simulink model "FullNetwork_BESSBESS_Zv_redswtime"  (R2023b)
settings: Solver=ode15s  StartTime=0.0  StopTime=140  RelTol=1e-3
PreLoadFcn:
  | Ts=50e-6;
model workspace (MAT data in the model file):
  Cf1 = 0.02
  Cf2 = 0.02
  Kffi1 = 0.9
  Kffi2 = 0.9
  Kffi3 = 0.9
  Kffv1 = 1
  Kffv2 = 1
  Kffv3 = 1
  Ki_cc1 = 5.9
  Ki_cc2 = 5.9
  Ki_cc3 = 5.9
  Ki_q1 = 0.0001
  Ki_q2 = 0.0001
  Ki_q3 = 0.0001
  Ki_vc1 = 150
  Ki_vc2 = 150
  Ki_vc3 = 150
  Kp_cc1 = 0.015
  Kp_cc2 = 0.015
  Kp_vc1 = 5
  Kp_vc2 = 5
  Kp_vc3 = 5
  Lf1 = 4.75e-06
  Lf2 = 4.75e-06
  Rf1 = 0.0005
  Rf2 = 0.0005
  Rf3 = 0.0005
  Rv1 = 0.0003169
  Rv2 = 0.0003169
  Snom1 = 100000000
  Snom2 = 100000000
  Vdc1 = 2000
  Vdc2 = 2000
  Vdc3 = 2000
  Xv1 = 0.0009509
  Xv2 = 0.0009509
  fnom1 = 50
  fnom2 = 50
  mp1 = 6.25e-08
  mp2 = 6.25e-08
  nq1 = 4.69166666667e-07
  nq2 = 4.69166666667e-07
  tau1 = 0.001
  tau2 = 0.001
  tau3 = 0.001
  vnom1 = 690
  vnom2 = 690
  vnom3 = 690
undefined symbols (not defined in the file or in its folder): Armidale, DiscIntNeverNeededParam, find_system, Gunnedah, Innerell, Ion, Lithium, Morree, Narrabri, Tamworth
libraries: spsThreePhaseBreakerLib x41, spsThreePhaseVIMeasurementLib x16, simulink_extras x16, spsThreePhaseSeriesRLCLoadLib x14, spsabctodq0Lib x12, spsThreePhaseTransformerTwoWindingsLib x11, slpidlib x8, spsLoadFlowBusLib x8, spsThreePhasePISectionLineLib x8, powerlib_extras x7, spsFirstOrderFilterLib x6, simulink x5
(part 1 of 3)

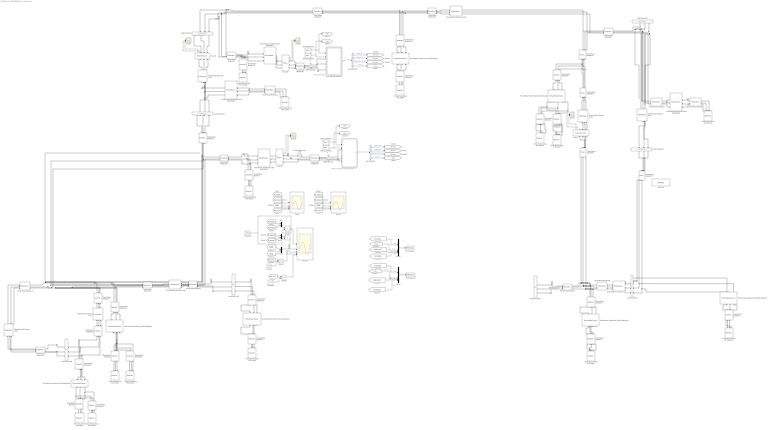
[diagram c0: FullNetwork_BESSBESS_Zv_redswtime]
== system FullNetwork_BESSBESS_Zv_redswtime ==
  note: Ts
  note: AC/DC conversion stage 80.0 MW
  note: Ts
  note: AC/DC conversion stage 80.0 MW
  B690 (690 V)1 : spsThreePhaseVIMeasurementLib/Three-Phase V-I Measurement  VoltageMeasurement=phase-to-ground  SetLabelV=on  LabelV=Vabc_B5751  Vpu=off  VpuLL=off  CurrentMeasurement=yes  SetLabelI=on  LabelI=Iabc_B5751  Ipu=off  Pbase=5*2e6/0.9  Vbase=575  OutputType=Complex  PhasorSimulation=off  PSBequivalent=0
  B690 (690 V)2 : spsThreePhaseVIMeasurementLib/Three-Phase V-I Measurement  VoltageMeasurement=phase-to-ground  SetLabelV=on  LabelV=Vabc_B5752  Vpu=off  VpuLL=off  CurrentMeasurement=yes  SetLabelI=on  LabelI=Iabc_B5752  Ipu=off  Pbase=5*2e6/0.9  Vbase=575  OutputType=Complex  PhasorSimulation=off  PSBequivalent=0
  B_grid1 : spsThreePhaseVIMeasurementLib/Three-Phase V-I Measurement  VoltageMeasurement=phase-to-ground  SetLabelV=off  LabelV=Vabc  Vpu=on  VpuLL=off  CurrentMeasurement=yes  SetLabelI=off  LabelI=Iabc  Ipu=on  Pbase=100e6  Vbase=132e3  OutputType=Complex  PhasorSimulation=off  PSBequivalent=0
  B_grid4 : spsThreePhaseVIMeasurementLib/Three-Phase V-I Measurement  VoltageMeasurement=phase-to-ground  SetLabelV=off  LabelV=Vabc  Vpu=on  VpuLL=off  CurrentMeasurement=yes  SetLabelI=off  LabelI=Iabc  Ipu=on  Pbase=100e6  Vbase=690  OutputType=Complex  PhasorSimulation=off  PSBequivalent=0
  B_grid5 : spsThreePhaseVIMeasurementLib/Three-Phase V-I Measurement  VoltageMeasurement=phase-to-ground  SetLabelV=off  LabelV=Vabc  Vpu=on  VpuLL=off  CurrentMeasurement=yes  SetLabelI=off  LabelI=Iabc  Ipu=on  Pbase=100e6  Vbase=690  OutputType=Complex  PhasorSimulation=off  PSBequivalent=0
  B_grid7 : spsThreePhaseVIMeasurementLib/Three-Phase V-I Measurement  VoltageMeasurement=phase-to-ground  SetLabelV=off  LabelV=Vabc  Vpu=on  VpuLL=off  CurrentMeasurement=yes  SetLabelI=off  LabelI=Iabc  Ipu=on  Pbase=100e6  Vbase=132e3  OutputType=Complex  PhasorSimulation=off  PSBequivalent=0
  Bus Selector1 : BusSelector  OutputSignals=Vabc_pcc,Iabc_pcc,Iabc_grid_conv_pu,Freq
  Bus Selector2 : BusSelector  OutputSignals=Vabc_pcc,Iabc_pcc,Iabc_grid_conv_pu,Freq
  Constant : Constant  Value=563
  Constant1 : Constant  Value=563
  Constant2 : Constant  Value=100e6
  Current Measurement2 : spsCurrentMeasurementLib/Current Measurement  PhasorSimulation=off  OutputType=Complex  PSBequivalent=0
  Divide{,1..3} (4 alike) : Product  Inputs=*/
  Grid forming inverter1 : Subsystem  LoadFcn=%find_system(gcs,'FollowLinks', 'on', 'LookUnderMasks', 'all');  mask(Grid forming inverter){Vnom=vnom1, fnom=fnom1, Pnom=Snom1, Lf=Lf1, Rf=Rf1, Cf=Cf1, Vdc_nom=Vdc1, Innerloops=Inner loops, Kp_cc=Kp_cc1, Ki_cc=Ki_cc1, Kffv=Kffv1, Kp_vc=Kp_vc1, Ki_vc=Ki_vc1, Kffi=Kffi1, Virtualimpedance=Virtual impedance, Rvir=Rv1, Lvir=Xv1, ControlType=Virtual Synchronous Machine, mp=mp1, nq=nq1, Ki_q=Ki_q1, tau=tau1, Ts=5e-5}
      mask prompts: Vnom "Grid-side converter nominal AC voltage (V):"; fnom "Grid frequency (Hz)"; Pnom "Nominal power (VA)"; Lf "Filter inductance (H)"; Rf "Filter resistance (Ω)"; Cf "Filter capacitor (F):"; Vdc_nom "Nominal DC bus voltage (V)"; Innerloops "Inner loops"; Kp_cc "Proportional gain of the current controller"; Ki_cc "Integral gain of the current controller"; Kffv "Voltage feed-forward"; Kp_vc "Proportional gain of the voltage controller"; Ki_vc "Integral gain of the voltage controller"; Kffi "Current feed-forward"; Virtualimpedance "Virtual impedance"; Rvir "Resistance of the virtual impedance"; Lvir "Inductance of the virtual impedance"; ControlType "Primary control"; mp "P - ω Droop coefficient"; nq "Q - V Droop coefficient"; Ki_q "Integral gain of the reactive power controller"; tau "Filter time constant (s)"; Ts "Sample time (s):"
      mask help: This block implements a model of a grid forming inverter with either droop or virtual synchronous generator control.
      mask init:
      | % Converters data
      | Q_filter=50;
      | 
      | % Controller data
      | Freq_filter=10000;   %Hz
      | Zeta_filter=0.707;
      | Mod_index_max=1.1;
      | T_speed=5;      %Speed reference time constant (s)
      | Iq_ref_limit_time_constant=0.3; %(s)
      | Current_reg_output_limit=1.1;   %(pu)
      | Var_reg_output_hi_limit=1.1;    %(pu)
      | Var_reg_output_low_limit=0.9;   %(pu)
      | Pitch_time_constant=0.01;       %(s)
      | Vf_limit=10;    %Field voltage limit (pu)
      | Freq_sawtooth=2000; %Hz, Boost converter
      | Freq_PWM=3000; %Hz, Inverter
      | Ts_snub=50e-6;  %Sample time to compute snubber resistance
  Grid forming inverter3 : Subsystem  LoadFcn=%find_system(gcs,'FollowLinks', 'on', 'LookUnderMasks', 'all');  mask(Grid forming inverter){Vnom=vnom2, fnom=fnom2, Pnom=Snom2, Lf=Lf2, Rf=Rf2, Cf=Cf2, Vdc_nom=Vdc2, Innerloops=Inner loops, Kp_cc=Kp_cc2, Ki_cc=Ki_cc2, Kffv=Kffv2, Kp_vc=Kp_vc2, Ki_vc=Ki_vc2, Kffi=Kffi2, Virtualimpedance=Virtual impedance, Rvir=Rv2, Lvir=Xv2, ControlType=Virtual Synchronous Machine, mp=mp2, nq=nq2, Ki_q=Ki_q2, tau=tau2, Ts=5e-5}
      mask prompts: Vnom "Grid-side converter nominal AC voltage (V):"; fnom "Grid frequency (Hz)"; Pnom "Nominal power (VA)"; Lf "Filter inductance (H)"; Rf "Filter resistance (Ω)"; Cf "Filter capacitor (F):"; Vdc_nom "Nominal DC bus voltage (V)"; Innerloops "Inner loops"; Kp_cc "Proportional gain of the current controller"; Ki_cc "Integral gain of the current controller"; Kffv "Voltage feed-forward"; Kp_vc "Proportional gain of the voltage controller"; Ki_vc "Integral gain of the voltage controller"; Kffi "Current feed-forward"; Virtualimpedance "Virtual impedance"; Rvir "Resistance of the virtual impedance"; Lvir "Inductance of the virtual impedance"; ControlType "Primary control"; mp "P - ω Droop coefficient"; nq "Q - V Droop coefficient"; Ki_q "Integral gain of the reactive power controller"; tau "Filter time constant (s)"; Ts "Sample time (s):"
      mask help: This block implements a model of a grid forming inverter with either droop or virtual synchronous generator control.
      mask init:
      | % Converters data
      | Q_filter=50;
      | 
      | % Controller data
      | Freq_filter=10000;   %Hz
      | Zeta_filter=0.707;
      | Mod_index_max=1.1;
      | T_speed=5;      %Speed reference time constant (s)
      | Iq_ref_limit_time_constant=0.3; %(s)
      | Current_reg_output_limit=1.1;   %(pu)
      | Var_reg_output_hi_limit=1.1;    %(pu)
      | Var_reg_output_low_limit=0.9;   %(pu)
      | Pitch_time_constant=0.01;       %(s)
      | Vf_limit=10;    %Field voltage limit (pu)
      | Freq_sawtooth=2000; %Hz, Boost converter
      | Freq_PWM=3000; %Hz, Inverter
      | Ts_snub=50e-6;  %Sample time to compute snubber resistance
  Load Flow Bus1 : spsLoadFlowBusLib/Load Flow Bus  LConnTagsString=a|b|c  RConnTagsString=a|b|c  Phases=ABC  Connectors=on both sides  ID=Innerell 132  Vbase=132e3  Vref=1  Vangle=0  VLF=1  VLFb=1  VLFc=1  angleLF=0  angleLFb=0  angleLFc=0
  Load Flow Bus11 : spsLoadFlowBusLib/Load Flow Bus  LConnTagsString=a|b|c  RConnTagsString=a|b|c  Phases=ABC  Connectors=on both sides  ID=Armidale 132  Vbase=132e3  Vref=1  Vangle=0  VLF=1  VLFb=1  VLFc=1  angleLF=0  angleLFb=0  angleLFc=0
  Load Flow Bus2 : spsLoadFlowBusLib/Load Flow Bus  LConnTagsString=a|b|c  RConnTagsString=a|b|c  Phases=ABC  Connectors=on both sides  ID=Innerell 132  Vbase=132e3  Vref=1  Vangle=0  VLF=1  VLFb=1  VLFc=1  angleLF=0  angleLFb=0  angleLFc=0
  Load Flow Bus3 : spsLoadFlowBusLib/Load Flow Bus  LConnTagsString=a|b|c  RConnTagsString=a|b|c  Phases=ABC  Connectors=on both sides  ID=Tamworth 132  Vbase=132e3  Vref=1  Vangle=0  VLF=1  VLFb=1  VLFc=1  angleLF=0  angleLFb=0  angleLFc=0
  Load Flow Bus6 : spsLoadFlowBusLib/Load Flow Bus  LConnTagsString=a|b|c  RConnTagsString=a|b|c  Phases=ABC  Connectors=on both sides  ID=Narrabri 132  Vbase=132e3  Vref=1  Vangle=0  VLF=1  VLFb=1  VLFc=1  angleLF=0  angleLFb=0  angleLFc=0
  Load Flow Bus7 : spsLoadFlowBusLib/Load Flow Bus  LConnTagsString=a|b|c  RConnTagsString=a|b|c  Phases=ABC  Connectors=on both sides  ID=Morree 132  Vbase=132e3  Vref=1  Vangle=0  VLF=1  VLFb=1  VLFc=1  angleLF=0  angleLFb=0  angleLFc=0
  Load Flow Bus8 : spsLoadFlowBusLib/Load Flow Bus  LConnTagsString=a|b|c  RConnTagsString=a|b|c  Phases=ABC  Connectors=on both sides  ID=Gunnedah 132  Vbase=132e3  Vref=1  Vangle=0  VLF=1  VLFb=1  VLFc=1  angleLF=0  angleLFb=0  angleLFc=0
  Load Flow Bus9 : spsLoadFlowBusLib/Load Flow Bus  LConnTagsString=a|b|c  RConnTagsString=a|b|c  Phases=ABC  Connectors=on both sides  ID=Glen Innes 132  Vbase=132e3  Vref=1  Vangle=0  VLF=1  VLFb=1  VLFc=1  angleLF=0  angleLFb=0  angleLFc=0
  Mux : Mux  Inputs=2
  Mux1 : Mux  Inputs=2
  Mux2 : Mux  Inputs=2
  Mux5 : Mux
  Mux6 : Mux
  Scope : Scope  NumInputPorts=4
  Scope1 : Scope  NumInputPorts=4
  Scope2 : Scope  NumInputPorts=5
  Scope{4,7..9} (4 alike) : Scope  NumInputPorts=2
  Stair Generator3 : spsStairGeneratorLib/Stair Generator  t=[0]  e=[0]  Ts=0
  Stair Generator4 : spsStairGeneratorLib/Stair Generator  t=[10]  e=[100]  Ts=0
  Stair Generator5 : spsStairGeneratorLib/Stair Generator  t=[0]  e=[0]  Ts=0
  Stair Generator6 : spsStairGeneratorLib/Stair Generator  t=[10]  e=[100]  Ts=0
  Three-Phase PI Section Line : spsThreePhasePISectionLineLib/Three-Phase PI Section Line  LConnTagsString=a|b|c  RConnTagsString=A|B|C  Length=100  Frequency=50  Resistances=[14.13/100 44.25/100]  Inductances=[0.0012/100 00.0036/100]  Capacitances=[ 0.0865e-5/100 0.0642e-5/100]
  Three-Phase PI Section Line10 : spsThreePhasePISectionLineLib/Three-Phase PI Section Line  LConnTagsString=a|b|c  RConnTagsString=A|B|C  Length=100  Frequency=50  Resistances=[ 22.63/100 50.7213/100]  Inductances=[ 0.1852/100 0.4654/100]  Capacitances=[ 0.1309e-5/100 0.0815e-5/100]
  Three-Phase PI Section Line2 : spsThreePhasePISectionLineLib/Three-Phase PI Section Line  LConnTagsString=a|b|c  RConnTagsString=A|B|C  Length=100  Frequency=50  Resistances=[14.13/100 44.25/100]  Inductances=[0.0012/100 00.0036/100]  Capacitances=[ 0.0865e-5/100 0.0642e-5/100]
  Three-Phase PI Section Line3 : spsThreePhasePISectionLineLib/Three-Phase PI Section Line  LConnTagsString=a|b|c  RConnTagsString=A|B|C  Length=100  Frequency=50  Resistances=[13.7127/100 32.2867/100]  Inductances="[0.0836/100  0.2361/100]"  Capacitances=[ 0.0722e-5/100 0.0450e-5/100]
  Three-Phase PI Section Line4 : spsThreePhasePISectionLineLib/Three-Phase PI Section Line  LConnTagsString=a|b|c  RConnTagsString=A|B|C  Length=100  Frequency=50  Resistances=[ 25.7875/100 79.97/100]  Inductances=[ 0.2286/100 0.5/100]  Capacitances=[0.1603e-5/100 0.1188e-5/100]
  Three-Phase PI Section Line6 : spsThreePhasePISectionLineLib/Three-Phase PI Section Line  LConnTagsString=a|b|c  RConnTagsString=A|B|C  Length=100  Frequency=50  Resistances=[ 21.08/100 51.92/100]  Inductances="[ 0.1465/100  0.4184/100]"  Capacitances=[ 0.0918e-5/100 0.0698e-5/100]
  Three-Phase PI Section Line7 : spsThreePhasePISectionLineLib/Three-Phase PI Section Line  LConnTagsString=a|b|c  RConnTagsString=A|B|C  Length=100  Frequency=50  Resistances=[13.7127/100 32.2867/100]  Inductances="[0.0836/100  0.2361/100]"  Capacitances=[ 0.0722e-5/100 0.0450e-5/100]
  Three-Phase PI Section Line9 : spsThreePhasePISectionLineLib/Three-Phase PI Section Line  LConnTagsString=a|b|c  RConnTagsString=A|B|C  Length=100  Frequency=50  Resistances=[ 16.37/100 50.8781/100]  Inductances="[ 0.1465/100  0.4262/100]"  Capacitances=[ 0.1e-5/100 0.0724e-5/100]
  Three-Phase Series RLC Load1 : spsThreePhaseSeriesRLCLoadLib/Three-Phase Series RLC Load  LConnTagsString=A|B|C  Configuration=Y (grounded)  NominalVoltage=(66000)*1  Vabc=[1e3 1e3 1e3]  Vabcp=[1e3 1e3 1e3]  NominalFrequency=50  UnbalancedPower=off  ActivePower=20e6  InductivePower=10e6  CapacitivePower=0  Pabc=[10e3 9e3 11e3]  QLabc=[100 90 110]  QCabc=[100 90 110]  Pabcp=[10e3 9e3 11e3]  QLabcp=[100 90 110]  QCabcp=[100 90 110]  Measurements=None  LoadType=constant PQ
  Three-Phase Series RLC Load10 : spsThreePhaseSeriesRLCLoadLib/Three-Phase Series RLC Load  LConnTagsString=A|B|C  Configuration=Y (grounded)  NominalVoltage=(132000)*1  Vabc=[1e3 1e3 1e3]  Vabcp=[1e3 1e3 1e3]  NominalFrequency=50  UnbalancedPower=off  ActivePower=5e6  InductivePower=3e6  CapacitivePower=0  Pabc=[10e3 9e3 11e3]  QLabc=[100 90 110]  QCabc=[100 90 110]  Pabcp=[10e3 9e3 11e3]  QLabcp=[100 90 110]  QCabcp=[100 90 110]  Measurements=None  LoadType=constant PQ
  Three-Phase Series RLC Load11 : spsThreePhaseSeriesRLCLoadLib/Three-Phase Series RLC Load  LConnTagsString=A|B|C  Configuration=Y (grounded)  NominalVoltage=66000  Vabc=[1e3 1e3 1e3]  Vabcp=[1e3 1e3 1e3]  NominalFrequency=50  UnbalancedPower=off  ActivePower=5e6  InductivePower=1e6  CapacitivePower=0  Pabc=[10e3 9e3 11e3]  QLabc=[100 90 110]  QCabc=[100 90 110]  Pabcp=[10e3 9e3 11e3]  QLabcp=[100 90 110]  QCabcp=[100 90 110]  Measurements=None  LoadType=constant PQ
  Three-Phase Series RLC Load12 : spsThreePhaseSeriesRLCLoadLib/Three-Phase Series RLC Load  LConnTagsString=A|B|C  Configuration=Y (grounded)  NominalVoltage=66000  Vabc=[1e3 1e3 1e3]  Vabcp=[1e3 1e3 1e3]  NominalFrequency=50  UnbalancedPower=off  ActivePower=7e6  InductivePower=2e6  CapacitivePower=0  Pabc=[10e3 9e3 11e3]  QLabc=[100 90 110]  QCabc=[100 90 110]  Pabcp=[10e3 9e3 11e3]  QLabcp=[100 90 110]  QCabcp=[100 90 110]  Measurements=None  LoadType=constant PQ
  Three-Phase Series RLC Load13 : spsThreePhaseSeriesRLCLoadLib/Three-Phase Series RLC Load  LConnTagsString=A|B|C  Configuration=Y (grounded)  NominalVoltage=66000  Vabc=[1e3 1e3 1e3]  Vabcp=[1e3 1e3 1e3]  NominalFrequency=50  UnbalancedPower=off  ActivePower=12500  InductivePower=0  CapacitivePower=0  Pabc=[10e3 9e3 11e3]  QLabc=[100 90 110]  QCabc=[100 90 110]  Pabcp=[10e3 9e3 11e3]  QLabcp=[100 90 110]  QCabcp=[100 90 110]  Measurements=None  LoadType=constant PQ
  Three-Phase Series RLC Load14 : spsThreePhaseSeriesRLCLoadLib/Three-Phase Series RLC Load  LConnTagsString=A|B|C  Configuration=Y (grounded)  NominalVoltage=66000  Vabc=[1e3 1e3 1e3]  Vabcp=[1e3 1e3 1e3]  NominalFrequency=50  UnbalancedPower=off  ActivePower=5e6  InductivePower=1.5e6  CapacitivePower=0  Pabc=[10e3 9e3 11e3]  QLabc=[100 90 110]  QCabc=[100 90 110]  Pabcp=[10e3 9e3 11e3]  QLabcp=[100 90 110]  QCabcp=[100 90 110]  Measurements=None  LoadType=constant PQ
  Three-Phase Series RLC Load2 : spsThreePhaseSeriesRLCLoadLib/Three-Phase Series RLC Load  LConnTagsString=A|B|C  Configuration=Y (grounded)  NominalVoltage=66000  Vabc=[1e3 1e3 1e3]  Vabcp=[1e3 1e3 1e3]  NominalFrequency=50  UnbalancedPower=off  ActivePower=10e6  InductivePower=4e6  CapacitivePower=0  Pabc=[10e3 9e3 11e3]  QLabc=[100 90 110]  QCabc=[100 90 110]  Pabcp=[10e3 9e3 11e3]  QLabcp=[100 90 110]  QCabcp=[100 90 110]  Measurements=None  LoadType=constant PQ
  Three-Phase Series RLC Load3 : spsThreePhaseSeriesRLCLoadLib/Three-Phase Series RLC Load  LConnTagsString=A|B|C  Configuration=Y (grounded)  NominalVoltage=66000  Vabc=[1e3 1e3 1e3]  Vabcp=[1e3 1e3 1e3]  NominalFrequency=50  UnbalancedPower=off  ActivePower=5e6  InductivePower=1.5e6  CapacitivePower=0  Pabc=[10e3 9e3 11e3]  QLabc=[100 90 110]  QCabc=[100 90 110]  Pabcp=[10e3 9e3 11e3]  QLabcp=[100 90 110]  QCabcp=[100 90 110]  Measurements=None  LoadType=constant PQ
  Three-Phase Series RLC Load4 : spsThreePhaseSeriesRLCLoadLib/Three-Phase Series RLC Load  LConnTagsString=A|B|C  Configuration=Y (grounded)  NominalVoltage=66000  Vabc=[1e3 1e3 1e3]  Vabcp=[1e3 1e3 1e3]  NominalFrequency=50  UnbalancedPower=off  ActivePower=0.10e6  InductivePower=0.4e6  CapacitivePower=0  Pabc=[10e3 9e3 11e3]  QLabc=[100 90 110]  QCabc=[100 90 110]  Pabcp=[10e3 9e3 11e3]  QLabcp=[100 90 110]  QCabcp=[100 90 110]  Measurements=None  LoadType=constant PQ
  Three-Phase Series RLC Load5 : spsThreePhaseSeriesRLCLoadLib/Three-Phase Series RLC Load  LConnTagsString=A|B|C  Configuration=Y (grounded)  NominalVoltage=(66000)*1  Vabc=[1e3 1e3 1e3]  Vabcp=[1e3 1e3 1e3]  NominalFrequency=50  UnbalancedPower=off  ActivePower=10e6  InductivePower=3e6  CapacitivePower=0  Pabc=[10e3 9e3 11e3]  QLabc=[100 90 110]  QCabc=[100 90 110]  Pabcp=[10e3 9e3 11e3]  QLabcp=[100 90 110]  QCabcp=[100 90 110]  Measurements=None  LoadType=constant PQ
  Three-Phase Series RLC Load6 : spsThreePhaseSeriesRLCLoadLib/Three-Phase Series RLC Load  LConnTagsString=A|B|C  Configuration=Y (grounded)  NominalVoltage=66000  Vabc=[1e3 1e3 1e3]  Vabcp=[1e3 1e3 1e3]  NominalFrequency=50  UnbalancedPower=off  ActivePower=7e6  InductivePower=2e6  CapacitivePower=0  Pabc=[10e3 9e3 11e3]  QLabc=[100 90 110]  QCabc=[100 90 110]  Pabcp=[10e3 9e3 11e3]  QLabcp=[100 90 110]  QCabcp=[100 90 110]  Measurements=None  LoadType=constant PQ
  Three-Phase Series RLC Load7 : spsThreePhaseSeriesRLCLoadLib/Three-Phase Series RLC Load  LConnTagsString=A|B|C  Configuration=Y (grounded)  NominalVoltage=66000  Vabc=[1e3 1e3 1e3]  Vabcp=[1e3 1e3 1e3]  NominalFrequency=50  UnbalancedPower=off  ActivePower=5e6  InductivePower=1e6  CapacitivePower=0  Pabc=[10e3 9e3 11e3]  QLabc=[100 90 110]  QCabc=[100 90 110]  Pabcp=[10e3 9e3 11e3]  QLabcp=[100 90 110]  QCabcp=[100 90 110]  Measurements=None  LoadType=constant PQ
  Three-Phase Series RLC Load8 : spsThreePhaseSeriesRLCLoadLib/Three-Phase Series RLC Load  LConnTagsString=A|B|C  Configuration=Y (grounded)  NominalVoltage=66000  Vabc=[1e3 1e3 1e3]  Vabcp=[1e3 1e3 1e3]  NominalFrequency=50  UnbalancedPower=off  ActivePower=10e6  InductivePower=5e6  CapacitivePower=0  Pabc=[10e3 9e3 11e3]  QLabc=[100 90 110]  QCabc=[100 90 110]  Pabcp=[10e3 9e3 11e3]  QLabcp=[100 90 110]  QCabcp=[100 90 110]  Measurements=None  LoadType=constant PQ
  Three-Phase Series RLC Load9 : spsThreePhaseSeriesRLCLoadLib/Three-Phase Series RLC Load  LConnTagsString=A|B|C  Configuration=Y (grounded)  NominalVoltage=(132000)*1  Vabc=[1e3 1e3 1e3]  Vabcp=[1e3 1e3 1e3]  NominalFrequency=50  UnbalancedPower=off  ActivePower=5e6  InductivePower=4e6  CapacitivePower=0  Pabc=[10e3 9e3 11e3]  QLabc=[100 90 110]  QCabc=[100 90 110]  Pabcp=[10e3 9e3 11e3]  QLabcp=[100 90 110]  QCabcp=[100 90 110]  Measurements=None  LoadType=constant PQ
  Three-Phase Transformer (Two Windings)1 : spsThreePhaseTransformerTwoWindingsLib/Three-Phase Transformer (Two Windings)  Winding1Connection=Yg  Winding2Connection=Yg  CoreType=Three single-phase transformers  SetSaturation=off  Hysteresis=off  DataFile='hysteresis'  SetInitialFlux=off  Measurements=None  UNITS=pu  NominalPower=[ 120e6 , 50 ]  Winding1=[ 66e3 , 0 , 0.09 ]  Winding2=[ 132e3 ,0 , 0.09 ]  Rm=500  Lm=500  L0=0.5  Saturation=[ 0,0 ; 0.0024,1.2 ; 1.0,1.52 ]  InitialFluxes=[0 0 0]  BreakLoop=off  DiscreteSolver=Trapezoidal iterative  DataType=off  TransfoNumber=1
  Three-Phase Transformer (Two Windings)10 : spsThreePhaseTransformerTwoWindingsLib/Three-Phase Transformer (Two Windings)  Winding1Connection=Yg  Winding2Connection=Yg  CoreType=Three single-phase transformers  SetSaturation=off  Hysteresis=off  DataFile='hysteresis'  SetInitialFlux=off  Measurements=None  UNITS=pu  NominalPower=[ 120e6 , 50 ]  Winding1=[ 132e3 , 0 , 0.1 ]  Winding2=[ 66e3 , 0 , 0.1 ]  Rm=500  Lm=500  L0=0.5  Saturation=[ 0,0 ; 0.0024,1.2 ; 1.0,1.52 ]  InitialFluxes=[0 0 0]  BreakLoop=off  DiscreteSolver=Trapezoidal iterative  DataType=off  TransfoNumber=1
  Three-Phase Transformer (Two Windings)11 : spsThreePhaseTransformerTwoWindingsLib/Three-Phase Transformer (Two Windings)  Winding1Connection=Yg  Winding2Connection=Yg  CoreType=Three single-phase transformers  SetSaturation=off  Hysteresis=off  DataFile='hysteresis'  SetInitialFlux=off  Measurements=None  UNITS=pu  NominalPower=[ 120e6 , 50 ]  Winding1=[ 132e3 , 0 , 0.1 ]  Winding2=[ 66e3 , 0 , 0.1 ]  Rm=500  Lm=500  L0=0.5  Saturation=[ 0,0 ; 0.0024,1.2 ; 1.0,1.52 ]  InitialFluxes=[0 0 0]  BreakLoop=off  DiscreteSolver=Trapezoidal iterative  DataType=off  TransfoNumber=1
  Three-Phase Transformer (Two Windings)2 : spsThreePhaseTransformerTwoWindingsLib/Three-Phase Transformer (Two Windings)  Winding1Connection=Yg  Winding2Connection=Yg  CoreType=Three single-phase transformers  SetSaturation=off  Hysteresis=off  DataFile='hysteresis'  SetInitialFlux=off  Measurements=None  UNITS=pu  NominalPower=[ 100e6 , 50 ]  Winding1=[66e3 , 0.002 , 0.08 ]  Winding2=[ 132e3 , 0.002 , 0.08 ]  Rm=500  Lm=500  L0=0.5  Saturation=[ 0,0 ; 0.0024,1.2 ; 1.0,1.52 ]  InitialFluxes=[0 0 0]  BreakLoop=off  DiscreteSolver=Trapezoidal iterative  DataType=off  TransfoNumber=1
  Three-Phase Transformer (Two Windings)3 : spsThreePhaseTransformerTwoWindingsLib/Three-Phase Transformer (Two Windings)  Winding1Connection=Yg  Winding2Connection=Yg  CoreType=Three single-phase transformers  SetSaturation=off  Hysteresis=off  DataFile='hysteresis'  SetInitialFlux=off  Measurements=None  UNITS=pu  NominalPower=[ 180e6 , 50 ]  Winding1=[ 132e3 , 0 , 0.06 ]  Winding2=[ 66e3 , 0, 0.06 ]  Rm=500  Lm=500  L0=0.5  Saturation=[ 0,0 ; 0.0024,1.2 ; 1.0,1.52 ]  InitialFluxes=[0 0 0]  BreakLoop=off  DiscreteSolver=Trapezoidal iterative  DataType=off  TransfoNumber=1
  Three-Phase Transformer (Two Windings)4 : spsThreePhaseTransformerTwoWindingsLib/Three-Phase Transformer (Two Windings)  Winding1Connection=Yg  Winding2Connection=Yg  CoreType=Three-limb core (core-type)  SetSaturation=off  Hysteresis=off  DataFile='hysteresis'  SetInitialFlux=on  Measurements=All measurements (V I Fluxes)  UNITS=pu  NominalPower=[ 100e6 , 50 ]  Winding1=[132e3 , 0.002 , 0.08 ]  Winding2=[ 690 , 0.002 , 0.08 ]  Rm=500  Lm=500  L0=0.5  Saturation=[ 0,0 ; 0.0024,1.2 ; 1.0,1.52 ]  InitialFluxes=[-0.7 0 0.7]  BreakLoop=off  DiscreteSolver=Trapezoidal robust  DataType=off  TransfoNumber=1
  Three-Phase Transformer (Two Windings)5 : spsThreePhaseTransformerTwoWindingsLib/Three-Phase Transformer (Two Windings)  Winding1Connection=Yg  Winding2Connection=Yg  CoreType=Three-limb core (core-type)  SetSaturation=off  Hysteresis=off  DataFile='hysteresis'  SetInitialFlux=on  Measurements=All measurements (V I Fluxes)  UNITS=pu  NominalPower=[ 100e6 , 50 ]  Winding1=[132e3 , 0.002 , 0.08 ]  Winding2=[ 690 , 0.002 , 0.08 ]  Rm=500  Lm=500  L0=0.5  Saturation=[ 0,0 ; 0.0024,1.2 ; 1.0,1.52 ]  InitialFluxes=[-0.7 0 0.7]  BreakLoop=off  DiscreteSolver=Trapezoidal robust  DataType=off  TransfoNumber=1
  Three-Phase Transformer (Two Windings)6 : spsThreePhaseTransformerTwoWindingsLib/Three-Phase Transformer (Two Windings)  Winding1Connection=Yg  Winding2Connection=Yg  CoreType=Three single-phase transformers  SetSaturation=off  Hysteresis=off  DataFile='hysteresis'  SetInitialFlux=off  Measurements=None  UNITS=pu  NominalPower=[ 120e6 , 50 ]  Winding1=[ 132e3 , 0 , 0.09 ]  Winding2=[ 66e3 , 0 , 0.09 ]  Rm=500  Lm=500  L0=0.5  Saturation=[ 0,0 ; 0.0024,1.2 ; 1.0,1.52 ]  InitialFluxes=[0 0 0]  BreakLoop=off  DiscreteSolver=Trapezoidal iterative  DataType=off  TransfoNumber=1
  Three-Phase Transformer (Two Windings)7 : spsThreePhaseTransformerTwoWindingsLib/Three-Phase Transformer (Two Windings)  Winding1Connection=Yg  Winding2Connection=Yg  CoreType=Three single-phase transformers  SetSaturation=off  Hysteresis=off  DataFile='hysteresis'  SetInitialFlux=off  Measurements=None  UNITS=pu  NominalPower=[ 100e6 , 50 ]  Winding1=[ 66e3 , 0.002 , 0.08 ]  Winding2=[ 132e3 , 0.002 , 0.08 ]  Rm=500  Lm=500  L0=0.5  Saturation=[ 0,0 ; 0.0024,1.2 ; 1.0,1.52 ]  InitialFluxes=[0 0 0]  BreakLoop=off  DiscreteSolver=Trapezoidal iterative  DataType=off  TransfoNumber=1
  Three-Phase Transformer (Two Windings)8 : spsThreePhaseTransformerTwoWindingsLib/Three-Phase Transformer (Two Windings)  Winding1Connection=Yg  Winding2Connection=Yg  CoreType=Three single-phase transformers  SetSaturation=off  Hysteresis=off  DataFile='hysteresis'  SetInitialFlux=off  Measurements=None  UNITS=pu  NominalPower=[ 100e6 , 50 ]  Winding1=[ 66e3 , 0.002 , 0.08 ]  Winding2=[ 132e3 , 0.002 , 0.08 ]  Rm=500  Lm=500  L0=0.5  Saturation=[ 0,0 ; 0.0024,1.2 ; 1.0,1.52 ]  InitialFluxes=[0 0 0]  BreakLoop=off  DiscreteSolver=Trapezoidal iterative  DataType=off  TransfoNumber=1
  Three-Phase Transformer (Two Windings)9 : spsThreePhaseTransformerTwoWindingsLib/Three-Phase Transformer (Two Windings)  Winding1Connection=Yg  Winding2Connection=Yg  CoreType=Three single-phase transformers  SetSaturation=off  Hysteresis=off  DataFile='hysteresis'  SetInitialFlux=off  Measurements=None  UNITS=pu  NominalPower=[ 120e6 , 50 ]  Winding1=[ 132e3 , 0 , 0.05 ]  Winding2=[ 66e3 , 0 , 0.05 ]  Rm=500  Lm=500  L0=0.5  Saturation=[ 0,0 ; 0.0024,1.2 ; 1.0,1.52 ]  InitialFluxes=[0 0 0]  BreakLoop=off  DiscreteSolver=Trapezoidal iterative  DataType=off  TransfoNumber=1
  Three-Phase Breaker1 : spsThreePhaseBreakerLib/Three-Phase Breaker  InitialState=open  SwitchA=on  SwitchB=on  SwitchC=on  SwitchTimes=90  External=off  BreakerResistance=1e-10  SnubberResistance=1e10  SnubberCapacitance=inf  Measurements=None
  Three-Phase Breaker10 : spsThreePhaseBreakerLib/Three-Phase Breaker  InitialState=open  SwitchA=on  SwitchB=on  SwitchC=on  SwitchTimes=[2]  External=off  BreakerResistance=1e-10  SnubberResistance=1e10  SnubberCapacitance=inf  Measurements=None
  Three-Phase Breaker11 : spsThreePhaseBreakerLib/Three-Phase Breaker  InitialState=open  SwitchA=on  SwitchB=on  SwitchC=on  SwitchTimes=116  External=off  BreakerResistance=1e-10  SnubberResistance=1e10  SnubberCapacitance=inf  Measurements=None
  Three-Phase Breaker12 : spsThreePhaseBreakerLib/Three-Phase Breaker  InitialState=open  SwitchA=on  SwitchB=on  SwitchC=on  SwitchTimes=74  External=off  BreakerResistance=1e-10  SnubberResistance=1e10  SnubberCapacitance=inf  Measurements=None
  Three-Phase Breaker13 : spsThreePhaseBreakerLib/Three-Phase Breaker  InitialState=open  SwitchA=on  SwitchB=on  SwitchC=on  SwitchTimes=50  External=off  BreakerResistance=1e-10  SnubberResistance=1e10  SnubberCapacitance=inf  Measurements=None
  Three-Phase Breaker14 : spsThreePhaseBreakerLib/Three-Phase Breaker  InitialState=open  SwitchA=on  SwitchB=on  SwitchC=on  SwitchTimes=[26]  External=off  BreakerResistance=1e-10  SnubberResistance=1e10  SnubberCapacitance=inf  Measurements=None
  Three-Phase Breaker15 : spsThreePhaseBreakerLib/Three-Phase Breaker  InitialState=open  SwitchA=on  SwitchB=on  SwitchC=on  SwitchTimes=[2]  External=off  BreakerResistance=1e-10  SnubberResistance=1e10  SnubberCapacitance=inf  Measurements=None
  Three-Phase Breaker16 : spsThreePhaseBreakerLib/Three-Phase Breaker  InitialState=open  SwitchA=on  SwitchB=on  SwitchC=on  SwitchTimes=18  External=off  BreakerResistance=1e-10  SnubberResistance=1e10  SnubberCapacitance=inf  Measurements=None
  Three-Phase Breaker17 : spsThreePhaseBreakerLib/Three-Phase Breaker  InitialState=open  SwitchA=on  SwitchB=on  SwitchC=on  SwitchTimes=42  External=off  BreakerResistance=1e-10  SnubberResistance=1e10  SnubberCapacitance=inf  Measurements=None
  Three-Phase Breaker18 : spsThreePhaseBreakerLib/Three-Phase Breaker  InitialState=open  SwitchA=on  SwitchB=on  SwitchC=on  SwitchTimes=[26]  External=off  BreakerResistance=1e-10  SnubberResistance=1e10  SnubberCapacitance=inf  Measurements=None
  Three-Phase Breaker19 : spsThreePhaseBreakerLib/Three-Phase Breaker  InitialState=open  SwitchA=on  SwitchB=on  SwitchC=on  SwitchTimes=[120+58]  External=off  BreakerResistance=1e-10  SnubberResistance=1e10  SnubberCapacitance=inf  Measurements=None
  Three-Phase Breaker2 : spsThreePhaseBreakerLib/Three-Phase Breaker  InitialState=open  SwitchA=on  SwitchB=on  SwitchC=on  SwitchTimes=[34]  External=off  BreakerResistance=1e-10  SnubberResistance=1e10  SnubberCapacitance=inf  Measurements=None
  Three-Phase Breaker20 : spsThreePhaseBreakerLib/Three-Phase Breaker  InitialState=open  SwitchA=on  SwitchB=on  SwitchC=on  SwitchTimes=[26]  External=off  BreakerResistance=1e-10  SnubberResistance=1e10  SnubberCapacitance=inf  Measurements=None
  Three-Phase Breaker21 : spsThreePhaseBreakerLib/Three-Phase Breaker  InitialState=open  SwitchA=on  SwitchB=on  SwitchC=on  SwitchTimes=98  External=off  BreakerResistance=1e-10  SnubberResistance=1e10  SnubberCapacitance=inf  Measurements=None
  Three-Phase Breaker22 : spsThreePhaseBreakerLib/Three-Phase Breaker  InitialState=open  SwitchA=on  SwitchB=on  SwitchC=on  SwitchTimes=[120+42]  External=off  BreakerResistance=1e-10  SnubberResistance=1e10  SnubberCapacitance=inf  Measurements=None
  Three-Phase Breaker23 : spsThreePhaseBreakerLib/Three-Phase Breaker  InitialState=open  SwitchA=on  SwitchB=on  SwitchC=on  SwitchTimes=66  External=off  BreakerResistance=1e-10  SnubberResistance=1e10  SnubberCapacitance=inf  Measurements=None
  Three-Phase Breaker24 : spsThreePhaseBreakerLib/Three-Phase Breaker  InitialState=open  SwitchA=on  SwitchB=on  SwitchC=on  SwitchTimes=82  External=off  BreakerResistance=1e-10  SnubberResistance=1e10  SnubberCapacitance=inf  Measurements=None
  Three-Phase Breaker25 : spsThreePhaseBreakerLib/Three-Phase Breaker  InitialState=open  SwitchA=on  SwitchB=on  SwitchC=on  SwitchTimes=82  External=off  BreakerResistance=1e-10  SnubberResistance=1e10  SnubberCapacitance=inf  Measurements=None
  Three-Phase Breaker26 : spsThreePhaseBreakerLib/Three-Phase Breaker  InitialState=open  SwitchA=on  SwitchB=on  SwitchC=on  SwitchTimes=18  External=off  BreakerResistance=1e-10  SnubberResistance=1e10  SnubberCapacitance=inf  Measurements=None
  Three-Phase Breaker27 : spsThreePhaseBreakerLib/Three-Phase Breaker  InitialState=open  SwitchA=on  SwitchB=on  SwitchC=on  SwitchTimes=[120+42]  External=off  BreakerResistance=1e-10  SnubberResistance=1e10  SnubberCapacitance=inf  Measurements=None
  Three-Phase Breaker28 : spsThreePhaseBreakerLib/Three-Phase Breaker  InitialState=open  SwitchA=on  SwitchB=on  SwitchC=on  SwitchTimes=58  External=off  BreakerResistance=1e-10  SnubberResistance=1e10  SnubberCapacitance=inf  Measurements=None
  Three-Phase Breaker29 : spsThreePhaseBreakerLib/Three-Phase Breaker  InitialState=open  SwitchA=on  SwitchB=on  SwitchC=on  SwitchTimes=10+120  External=off  BreakerResistance=1e-10  SnubberResistance=1e10  SnubberCapacitance=inf  Measurements=None
  Three-Phase Breaker3 : spsThreePhaseBreakerLib/Three-Phase Breaker  InitialState=open  SwitchA=on  SwitchB=on  SwitchC=on  SwitchTimes=[2]  External=off  BreakerResistance=1e-10  SnubberResistance=1e10  SnubberCapacitance=inf  Measurements=None
  Three-Phase Breaker30 : spsThreePhaseBreakerLib/Three-Phase Breaker  InitialState=open  SwitchA=on  SwitchB=on  SwitchC=on  SwitchTimes=124  External=off  BreakerResistance=1e-10  SnubberResistance=1e10  SnubberCapacitance=inf  Measurements=None
  Three-Phase Breaker31 : spsThreePhaseBreakerLib/Three-Phase Breaker  InitialState=open  SwitchA=on  SwitchB=on  SwitchC=on  SwitchTimes=108  External=off  BreakerResistance=1e-10  SnubberResistance=1e10  SnubberCapacitance=inf  Measurements=None
  Three-Phase Breaker32 : spsThreePhaseBreakerLib/Three-Phase Breaker  InitialState=open  SwitchA=on  SwitchB=on  SwitchC=on  SwitchTimes=[65]  External=off  BreakerResistance=1e-10  SnubberResistance=1e10  SnubberCapacitance=inf  Measurements=None
  Three-Phase Breaker33 : spsThreePhaseBreakerLib/Three-Phase Breaker  InitialState=open  SwitchA=on  SwitchB=on  SwitchC=on  SwitchTimes=49  External=off  BreakerResistance=1e-10  SnubberResistance=1e10  SnubberCapacitance=inf  Measurements=None
  Three-Phase Breaker34 : spsThreePhaseBreakerLib/Three-Phase Breaker  InitialState=open  SwitchA=on  SwitchB=on  SwitchC=on  SwitchTimes=[33]  External=off  BreakerResistance=1e-10  SnubberResistance=1e10  SnubberCapacitance=inf  Measurements=None
  Three-Phase Breaker35 : spsThreePhaseBreakerLib/Three-Phase Breaker  InitialState=open  SwitchA=on  SwitchB=on  SwitchC=on  SwitchTimes=49  External=off  BreakerResistance=1e-10  SnubberResistance=1e10  SnubberCapacitance=inf  Measurements=None
  Three-Phase Breaker36 : spsThreePhaseBreakerLib/Three-Phase Breaker  InitialState=open  SwitchA=on  SwitchB=on  SwitchC=on  SwitchTimes=73  External=off  BreakerResistance=1e-10  SnubberResistance=1e10  SnubberCapacitance=inf  Measurements=None
  Three-Phase Breaker37 : spsThreePhaseBreakerLib/Three-Phase Breaker  InitialState=open  SwitchA=on  SwitchB=on  SwitchC=on  SwitchTimes=90  External=off  BreakerResistance=1e-10  SnubberResistance=1e10  SnubberCapacitance=inf  Measurements=None
  Three-Phase Breaker38 : spsThreePhaseBreakerLib/Three-Phase Breaker  InitialState=open  SwitchA=on  SwitchB=on  SwitchC=on  SwitchTimes=99  External=off  BreakerResistance=1e-10  SnubberResistance=1e10  SnubberCapacitance=inf  Measurements=None
  Three-Phase Breaker39 : spsThreePhaseBreakerLib/Three-Phase Breaker  InitialState=open  SwitchA=on  SwitchB=on  SwitchC=on  SwitchTimes=[34.5]  External=off  BreakerResistance=1e-10  SnubberResistance=1e10  SnubberCapacitance=inf  Measurements=None
  Three-Phase Breaker4 : spsThreePhaseBreakerLib/Three-Phase Breaker  InitialState=open  SwitchA=on  SwitchB=on  SwitchC=on  SwitchTimes=[66]  External=off  BreakerResistance=1e-10  SnubberResistance=1e10  SnubberCapacitance=inf  Measurements=None
  Three-Phase Breaker40 : spsThreePhaseBreakerLib/Three-Phase Breaker  InitialState=open  SwitchA=on  SwitchB=on  SwitchC=on  SwitchTimes=50.5  External=off  BreakerResistance=1e-10  SnubberResistance=1e10  SnubberCapacitance=inf  Measurements=None
  Three-Phase Breaker41 : spsThreePhaseBreakerLib/Three-Phase Breaker  InitialState=open  SwitchA=on  SwitchB=on  SwitchC=on  SwitchTimes=74.5  External=off  BreakerResistance=1e-10  SnubberResistance=1e10  SnubberCapacitance=inf  Measurements=None
  Three-Phase Breaker5 : spsThreePhaseBreakerLib/Three-Phase Breaker  InitialState=open  SwitchA=on  SwitchB=on  SwitchC=on  SwitchTimes=50  External=off  BreakerResistance=1e-10  SnubberResistance=1e10  SnubberCapacitance=inf  Measurements=None
  Three-Phase Breaker6 : spsThreePhaseBreakerLib/Three-Phase Breaker  InitialState=open  SwitchA=on  SwitchB=on  SwitchC=on  SwitchTimes=[58]  External=off  BreakerResistance=1e-10  SnubberResistance=1e10  SnubberCapacitance=inf  Measurements=None
  Three-Phase Breaker7 : spsThreePhaseBreakerLib/Three-Phase Breaker  InitialState=open  SwitchA=on  SwitchB=on  SwitchC=on  SwitchTimes=[120+10]  External=off  BreakerResistance=1e-10  SnubberResistance=1e10  SnubberCapacitance=inf  Measurements=None
  Three-Phase Breaker8 : spsThreePhaseBreakerLib/Three-Phase Breaker  InitialState=open  SwitchA=on  SwitchB=on  SwitchC=on  SwitchTimes=100  External=off  BreakerResistance=1e-10  SnubberResistance=1e10  SnubberCapacitance=inf  Measurements=None
  Three-Phase Breaker9 : spsThreePhaseBreakerLib/Three-Phase Breaker  InitialState=open  SwitchA=on  SwitchB=on  SwitchC=on  SwitchTimes=[15]  External=off  BreakerResistance=1e-10  SnubberResistance=1e10  SnubberCapacitance=inf  Measurements=None
  To Workspace : ToWorkspace  VariableName=BESSGFM1  SaveFormat=Timeseries  SampleTime=-1
  To Workspace1 : ToWorkspace  VariableName=BESSGFM2  SaveFormat=Timeseries  SampleTime=-1
  powergui : spspowerguiLib/powergui  SimulationMode=Discrete  SampleTime=5e-5  frequency=50  Iterations=50  frequencyindice=0  Pbase=100e6  ErrMax=1e-4  UnitsV=kV  UnitsW=MW  buscounter=0  FunctionMessages=off  echomessages=off  EnableUseOfTLC=on  CurrentSourceSwitches=off  DisableSnubberDevices=off  DisableRonSwitches=off  DisableVfSwitches=off  DisplayEquations=off  AutomaticDiscreteSolvers=off  SolverType=Tustin  Interpol=off  ExternalGateDelay=off  methode=off  Ts=0  x0status=blocks  SPID=off  SwTol=0  HookPort=off  NonlinearTolerance=1e-4  nMaxIteration=100  ContinueOnMaxIteration=off  RestoreLinks=warning  ResistiveCurrentMeasurement=off  Frange=[0:2:500]  Ylog=off  Xlog=on  ShowGrid=off  save=off  variable=ZData  structure=0  ZoomFFT=on  StartTime=0.0  cycles=1  DisplayStyle=1  fundamental=60  FreqAxis=off  MaxFrequency=1000  frequencyindicesteady=1  RmsSteady=1  display=off
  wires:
  Grid forming inverter3/1(m) -> Bus Selector2/1
  Bus Selector2/1 -> [Vabc_pcc2]  "<Vabc_pcc>"
  Bus Selector2/4 -> [Freq2]  "<Freq>"
  Bus Selector2/3 -> [Iabc_grid_conv_pu2]  "<Iabc_grid_conv_pu>"
  Stair Generator5/1 -> Grid forming inverter3/2(Pref_pu), [Pref2]
  Bus Selector2/2 -> [Iabc_pcc2]  "<Iabc_pcc>"
  Stair Generator6/1 -> Grid forming inverter3/1(Qref_pu), [Qref2]
  Stair Generator3/1 -> [Pref1], Grid forming inverter1/2(Pref_pu)
  Bus Selector1/2 -> [Iabc_pcc1]  "<Iabc_pcc>"
  Grid forming inverter1/1(m) -> Bus Selector1/1
  Stair Generator4/1 -> [Qref1], Grid forming inverter1/1(Qref_pu)
  Bus Selector1/3 -> [Iabc_grid_conv_pu1]  "<Iabc_grid_conv_pu>"
  Bus Selector1/1 -> [Vabc_pcc1]  "<Vabc_pcc>"
  Bus Selector1/4 -> [Freq1]  "<Freq>"
  [P_meas1] -> Scope/1
  [Q_meas1] -> Scope/2
  [Freq1] -> Scope/3
  [Vabc_pcc1] -> Scope/4
  [Q_meas2] -> Scope1/2
  [P_meas2] -> Scope1/1
  [Vabc_pcc2] -> Scope1/4
  [Freq2] -> Scope1/3
  [P_meas1] -> Mux/1
  [P_meas2] -> Mux/2
  [Q_meas1] -> Mux1/1
  [Q_meas2] -> Mux1/2
  [Freq1] -> Mux2/1
  [Freq2] -> Mux2/2
  Mux2/1 -> Scope2/3
  Mux/1 -> Divide/1
  Divide/1 -> Scope2/1
  Mux1/1 -> Divide1/1
  Divide1/1 -> Scope2/2
  [Vabc_pcc1] -> Divide2/1
  Divide2/1 -> Scope2/4
  [Vabc_pcc2] -> Divide3/1
  Divide3/1 -> Scope2/5
  Constant/1 -> Divide2/2
  Constant1/1 -> Divide3/2
  Constant2/1 -> Divide1/2, Divide/2
  Mux5/1 -> To Workspace/1
  [Vabc_pcc1] -> Mux5/3  "Freq"
  [P_meas1] -> Mux5/1  "Freq"
  [P_meas2] -> Mux6/1  "Freq"
  [Q_meas1] -> Mux5/4  "Freq"
  [Q_meas2] -> Mux6/4  "Freq"
  [Freq2] -> Mux6/2  "Freq"
  [Freq1] -> Mux5/2  "Freq"
  [Vabc_pcc2] -> Mux6/3  "Freq"
  Mux6/1 -> To Workspace1/1
  B_grid1/1 -> Scope4/1
  B_grid1/2 -> Scope4/2
  B_grid7/1 -> Scope7/1
  B_grid7/2 -> Scope7/2
  B_grid5/1 -> Scope8/1
  B_grid5/2 -> Scope8/2
  B_grid4/1 -> Scope9/1
  B_grid4/2 -> Scope9/2
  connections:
  Three-Phase Breaker37/RConn2 -- Three-Phase Breaker30/LConn2 -- Three-Phase Breaker25/LConn2 -- Three-Phase Breaker3/RConn2
  Three-Phase PI Section Line/RConn1 -- Load Flow Bus9/RConn1
  Three-Phase PI Section Line/RConn2 -- Load Flow Bus9/RConn2
  Three-Phase PI Section Line/RConn3 -- Load Flow Bus9/RConn3
  Three-Phase Breaker9/LConn1 -- Three-Phase Breaker16/LConn1 -- Three-Phase Breaker18/RConn1 -- Three-Phase Breaker27/RConn1 -- Three-Phase Breaker19/LConn1 -- Three-Phase Breaker33/RConn1
  Three-Phase Breaker27/RConn2 -- Three-Phase Breaker33/RConn2 -- Three-Phase Breaker19/LConn2 -- Three-Phase Breaker18/RConn2 -- Three-Phase Breaker16/LConn2 -- Three-Phase Breaker9/LConn2
  Three-Phase Breaker18/RConn3 -- Three-Phase Breaker33/RConn3 -- Three-Phase Breaker19/LConn3 -- Three-Phase Breaker27/RConn3 -- Three-Phase Breaker16/LConn3 -- Three-Phase Breaker9/LConn3
  Three-Phase Breaker22/LConn1 -- Three-Phase Breaker34/RConn1 -- Load Flow Bus8/LConn1
  Three-Phase Breaker22/LConn2 -- Three-Phase Breaker34/RConn2 -- Load Flow Bus8/LConn2
  Three-Phase Breaker22/LConn3 -- Three-Phase Breaker34/RConn3 -- Load Flow Bus8/LConn3
  Three-Phase Breaker9/RConn2 -- Load Flow Bus6/LConn2
  Three-Phase Breaker9/RConn3 -- Load Flow Bus6/LConn3
  Three-Phase Breaker9/RConn1 -- Load Flow Bus6/LConn1
  Three-Phase PI Section Line3/RConn1 -- Three-Phase Breaker20/LConn1
  Three-Phase PI Section Line3/RConn2 -- Three-Phase Breaker20/LConn2
  Three-Phase PI Section Line3/RConn3 -- Three-Phase Breaker20/LConn3
  Three-Phase Breaker37/RConn3 -- Three-Phase Breaker30/LConn3 -- Three-Phase Breaker3/RConn3 -- Three-Phase Breaker25/LConn3
  Three-Phase Breaker20/RConn1 -- Load Flow Bus8/RConn1
  Three-Phase Breaker20/RConn2 -- Load Flow Bus8/RConn2
  Load Flow Bus8/RConn3 -- Three-Phase Breaker20/RConn3
  Load Flow Bus6/RConn1 -- Three-Phase Transformer (Two Windings)6/LConn1 -- Three-Phase PI Section Line6/LConn1
  Load Flow Bus6/RConn2 -- Three-Phase Transformer (Two Windings)6/LConn2 -- Three-Phase PI Section Line6/LConn2
  Load Flow Bus6/RConn3 -- Three-Phase Transformer (Two Windings)6/LConn3 -- Three-Phase PI Section Line6/LConn3
  Three-Phase Breaker28/LConn1 -- Three-Phase Breaker35/RConn1 -- Three-Phase Breaker17/RConn1
  Three-Phase Breaker28/LConn2 -- Three-Phase Breaker35/RConn2 -- Three-Phase Breaker17/RConn2
  Three-Phase Breaker28/LConn3 -- Three-Phase Breaker35/RConn3 -- Three-Phase Breaker17/RConn3
  Load Flow Bus7/RConn1 -- Three-Phase Breaker26/LConn1 -- Three-Phase Breaker17/LConn1
  Load Flow Bus7/RConn2 -- Three-Phase Breaker26/LConn2 -- Three-Phase Breaker17/LConn2
  Load Flow Bus7/RConn3 -- Three-Phase Breaker26/LConn3 -- Three-Phase Breaker17/LConn3
  Three-Phase Breaker24/RConn2 -- Three-Phase Breaker36/RConn2 -- Three-Phase Breaker23/LConn2
  Three-Phase Breaker24/RConn3 -- Three-Phase Breaker36/RConn3 -- Three-Phase Breaker23/LConn3
  Three-Phase Breaker24/RConn1 -- Three-Phase Breaker36/RConn1 -- Three-Phase Breaker23/LConn1
  Load Flow Bus2/LConn1 -- Three-Phase Breaker38/LConn1 -- Three-Phase PI Section Line2/LConn1 -- Three-Phase Breaker21/RConn1
  Load Flow Bus2/LConn2 -- Three-Phase Breaker38/LConn2 -- Three-Phase PI Section Line2/LConn2 -- Three-Phase Breaker21/RConn2
  Load Flow Bus2/LConn3 -- Three-Phase Breaker38/LConn3 -- Three-Phase PI Section Line2/LConn3 -- Three-Phase Breaker21/RConn3
  Load Flow Bus1/LConn1 -- Three-Phase Breaker31/RConn1
  Load Flow Bus1/LConn3 -- Three-Phase Breaker31/RConn3
  Three-Phase Breaker30/LConn1 -- Three-Phase Breaker37/RConn1 -- Three-Phase Breaker25/LConn1 -- Three-Phase Breaker3/RConn1
  Load Flow Bus9/LConn2 -- Three-Phase Transformer (Two Windings)10/LConn3 -- Three-Phase Breaker31/LConn2
  Load Flow Bus9/LConn1 -- Three-Phase Transformer (Two Windings)10/LConn1 -- Three-Phase Breaker31/LConn1
  Load Flow Bus9/LConn3 -- Three-Phase Transformer (Two Windings)10/LConn2 -- Three-Phase Breaker31/LConn3
  Three-Phase Breaker8/RConn3 -- Three-Phase Series RLC Load2/LConn1
  Three-Phase Breaker8/RConn2 -- Three-Phase Series RLC Load2/LConn2
  Three-Phase Breaker8/RConn1 -- Three-Phase Series RLC Load2/LConn3
  Three-Phase Breaker14/RConn1 -- Three-Phase Series RLC Load5/LConn3
  Three-Phase Breaker14/RConn2 -- Three-Phase Series RLC Load5/LConn2
  Three-Phase Breaker14/RConn3 -- Three-Phase Series RLC Load5/LConn1
  Load Flow Bus1/LConn2 -- Three-Phase Breaker31/RConn2
  Load Flow Bus1/RConn1 -- Three-Phase PI Section Line2/RConn1
  Load Flow Bus1/RConn2 -- Three-Phase PI Section Line2/RConn2
  Load Flow Bus1/RConn3 -- Three-Phase PI Section Line2/RConn3
  Three-Phase PI Section Line4/LConn1 -- Three-Phase Breaker19/RConn1
  Three-Phase PI Section Line4/LConn2 -- Three-Phase Breaker19/RConn2
  Three-Phase PI Section Line4/LConn3 -- Three-Phase Breaker19/RConn3
  Three-Phase PI Section Line4/RConn1 -- Three-Phase Breaker6/LConn1
  Three-Phase PI Section Line4/RConn2 -- Three-Phase Breaker6/LConn2
  Three-Phase PI Section Line4/RConn3 -- Three-Phase Breaker6/LConn3
  Three-Phase Breaker6/RConn1 -- Load Flow Bus3/RConn1
  Three-Phase Breaker6/RConn2 -- Load Flow Bus3/RConn2
  Three-Phase Breaker6/RConn3 -- Load Flow Bus3/RConn3
  B690 (690 V)2/RConn1 -- Grid forming inverter3/LConn1
  B690 (690 V)2/RConn3 -- Grid forming inverter3/LConn3
  B690 (690 V)2/RConn2 -- Grid forming inverter3/LConn2
  Three-Phase Transformer (Two Windings)5/RConn1 -- B_grid5/LConn1
  Three-Phase Transformer (Two Windings)5/RConn2 -- B_grid5/LConn2
  Three-Phase Transformer (Two Windings)5/RConn3 -- B_grid5/LConn3
  Three-Phase Breaker10/RConn1 -- B690 (690 V)2/LConn1
  Three-Phase Breaker10/RConn2 -- B690 (690 V)2/LConn2
  Three-Phase Breaker10/RConn3 -- B690 (690 V)2/LConn3
  Three-Phase PI Section Line7/RConn1 -- Three-Phase Breaker22/RConn1
  Three-Phase PI Section Line7/RConn2 -- Three-Phase Breaker22/RConn2
  Three-Phase PI Section Line7/RConn3 -- Three-Phase Breaker22/RConn3
  Three-Phase Breaker18/LConn1 -- Three-Phase PI Section Line3/LConn1
  Three-Phase Breaker18/LConn2 -- Three-Phase PI Section Line3/LConn2
  Three-Phase Breaker18/LConn3 -- Three-Phase PI Section Line3/LConn3
  Three-Phase Breaker10/LConn1 -- B_grid5/RConn1
  Three-Phase Breaker10/LConn2 -- B_grid5/RConn2
  Three-Phase Breaker3/LConn1 -- Load Flow Bus11/LConn1
  Three-Phase Breaker3/LConn2 -- Load Flow Bus11/LConn2
  Three-Phase Breaker3/LConn3 -- Load Flow Bus11/LConn3
  B_grid4/RConn1 -- Current Measurement2/LConn1
  B690 (690 V)1/LConn1 -- Three-Phase Breaker15/RConn1
  Three-Phase Breaker16/RConn1 -- Three-Phase Breaker7/RConn1 -- Three-Phase Transformer (Two Windings)4/LConn1
  Current Measurement2/RConn1 -- Three-Phase Breaker15/LConn1
  Three-Phase Breaker16/RConn3 -- Three-Phase Breaker7/RConn3 -- Three-Phase Transformer (Two Windings)4/LConn3
  Grid forming inverter1/LConn1 -- B690 (690 V)1/RConn1
  Three-Phase Transformer (Two Windings)4/RConn1 -- B_grid4/LConn1
  B690 (690 V)1/LConn2 -- Three-Phase Breaker15/RConn2
  Grid forming inverter1/LConn2 -- B690 (690 V)1/RConn2
  B_grid4/RConn3 -- Three-Phase Breaker15/LConn3
  Three-Phase Transformer (Two Windings)4/RConn3 -- B_grid4/LConn3
  Three-Phase Breaker16/RConn2 -- Three-Phase Breaker7/RConn2 -- Three-Phase Transformer (Two Windings)4/LConn2
  Grid forming inverter1/LConn3 -- B690 (690 V)1/RConn3
  B_grid4/RConn2 -- Three-Phase Breaker15/LConn2
  B690 (690 V)1/LConn3 -- Three-Phase Breaker15/RConn3
  Three-Phase Transformer (Two Windings)4/RConn2 -- B_grid4/LConn2
  Three-Phase Breaker2/LConn3 -- Three-Phase Series RLC Load7/LConn3
  Three-Phase Breaker2/LConn2 -- Three-Phase Series RLC Load7/LConn2
  Three-Phase Breaker2/LConn1 -- Three-Phase Series RLC Load7/LConn1
  Three-Phase Breaker4/LConn1 -- Three-Phase Series RLC Load8/LConn1
  Three-Phase Breaker4/LConn2 -- Three-Phase Series RLC Load8/LConn2
  Three-Phase Breaker4/LConn3 -- Three-Phase Series RLC Load8/LConn3
  Three-Phase Breaker7/LConn1 -- Three-Phase Series RLC Load9/LConn1
  Three-Phase Breaker7/LConn2 -- Three-Phase Series RLC Load9/LConn2
  Three-Phase Breaker7/LConn3 -- Three-Phase Series RLC Load9/LConn3
  Three-Phase Breaker5/LConn1 -- Three-Phase Series RLC Load6/LConn1
  Three-Phase Breaker5/LConn2 -- Three-Phase Series RLC Load6/LConn2
  Three-Phase Breaker5/LConn3 -- Three-Phase Series RLC Load6/LConn3
  Three-Phase Breaker26/RConn2 -- Three-Phase Breaker29/RConn2 -- Three-Phase Transformer (Two Windings)5/LConn2
  Three-Phase Breaker26/RConn1 -- Three-Phase Breaker29/RConn1 -- Three-Phase Transformer (Two Windings)5/LConn1
  Three-Phase Breaker26/RConn3 -- Three-Phase Breaker29/RConn3 -- Three-Phase Transformer (Two Windings)5/LConn3
  Three-Phase Breaker29/LConn2 -- Three-Phase Series RLC Load10/LConn2
  Three-Phase Breaker29/LConn3 -- Three-Phase Series RLC Load10/LConn3
  Three-Phase Breaker28/RConn2 -- Three-Phase PI Section Line10/RConn2
  Three-Phase Breaker28/RConn1 -- Three-Phase PI Section Line10/RConn1
  Three-Phase Breaker28/RConn3 -- Three-Phase PI Section Line10/RConn3
  Three-Phase Breaker24/LConn1 -- Three-Phase PI Section Line9/LConn1
  Three-Phase Breaker24/LConn2 -- Three-Phase PI Section Line9/LConn2
  Three-Phase Breaker24/LConn3 -- Three-Phase PI Section Line9/LConn3
  Three-Phase Breaker30/RConn2 -- Three-Phase PI Section Line/LConn2
  Three-Phase Breaker30/RConn1 -- Three-Phase PI Section Line/LConn1
  Three-Phase Breaker30/RConn3 -- Three-Phase PI Section Line/LConn3
  Three-Phase Breaker10/LConn3 -- B_grid5/RConn3
  Three-Phase Series RLC Load10/LConn1 -- Three-Phase Breaker29/LConn1
  Three-Phase PI Section Line6/RConn1 -- B_grid1/LConn1
  Three-Phase PI Section Line6/RConn2 -- B_grid1/LConn2
  Three-Phase PI Section Line6/RConn3 -- B_grid1/LConn3
  B_grid1/RConn1 -- Load Flow Bus7/LConn1
  B_grid1/RConn2 -- Load Flow Bus7/LConn2
  B_grid1/RConn3 -- Load Flow Bus7/LConn3
  Three-Phase Breaker21/LConn1 -- Three-Phase PI Section Line10/LConn1 -- Three-Phase Breaker23/RConn1
  Three-Phase Breaker21/LConn2 -- Three-Phase PI Section Line10/LConn2 -- Three-Phase Breaker23/RConn2
  Three-Phase Breaker21/LConn3 -- Three-Phase PI Section Line10/LConn3 -- Three-Phase Breaker23/RConn3
  Three-Phase PI Section Line9/RConn1 -- B_grid7/RConn1
  Three-Phase PI Section Line9/RConn2 -- B_grid7/RConn2
  Three-Phase PI Section Line9/RConn3 -- B_grid7/RConn3
  B_grid7/LConn1 -- Three-Phase Breaker25/RConn1
  B_grid7/LConn2 -- Three-Phase Breaker25/RConn2
  B_grid7/LConn3 -- Three-Phase Breaker25/RConn3
  Three-Phase Breaker27/LConn1 -- Three-Phase PI Section Line7/LConn1
  Three-Phase Breaker27/LConn2 -- Three-Phase PI Section Line7/LConn2
  Three-Phase Breaker27/LConn3 -- Three-Phase PI Section Line7/LConn3
  Three-Phase Transformer (Two Windings)2/LConn1 -- Three-Phase Breaker40/RConn1 -- Three-Phase Breaker5/RConn1
  Three-Phase Transformer (Two Windings)2/LConn2 -- Three-Phase Breaker40/RConn2 -- Three-Phase Breaker5/RConn2
  Three-Phase Transformer (Two Windings)2/LConn3 -- Three-Phase Breaker40/RConn3 -- Three-Phase Breaker5/RConn3
  Three-Phase Breaker2/RConn1 -- Three-Phase Breaker39/RConn1 -- Three-Phase Transformer (Two Windings)1/LConn1
  Three-Phase Breaker2/RConn2 -- Three-Phase Breaker39/RConn2 -- Three-Phase Transformer (Two Windings)1/LConn2
  Three-Phase Breaker2/RConn3 -- Three-Phase Breaker39/RConn3 -- Three-Phase Transformer (Two Windings)1/LConn3
  Three-Phase Transformer (Two Windings)6/RConn1 -- Three-Phase Breaker14/LConn1
  Three-Phase Transformer (Two Windings)6/RConn2 -- Three-Phase Breaker14/LConn2
  Three-Phase Transformer (Two Windings)6/RConn3 -- Three-Phase Breaker14/LConn3
  Three-Phase Breaker8/LConn2 -- Three-Phase Transformer (Two Windings)9/RConn2
  Three-Phase Breaker8/LConn1 -- Three-Phase Transformer (Two Windings)9/RConn1
  Three-Phase Breaker8/LConn3 -- Three-Phase Transformer (Two Windings)9/RConn3
  Three-Phase Transformer (Two Windings)10/RConn2 -- Three-Phase Breaker11/LConn2
  Three-Phase Transformer (Two Windings)10/RConn1 -- Three-Phase Breaker11/LConn1
  Three-Phase Transformer (Two Windings)10/RConn3 -- Three-Phase Breaker11/LConn3
  Three-Phase Breaker32/RConn1 -- Load Flow Bus3/LConn1
  Three-Phase Breaker32/RConn2 -- Load Flow Bus3/LConn2
  Three-Phase Breaker32/RConn3 -- Load Flow Bus3/LConn3
  Three-Phase Breaker33/LConn1 -- Three-Phase Transformer (Two Windings)2/RConn1
  Three-Phase Breaker33/LConn2 -- Three-Phase Transformer (Two Windings)2/RConn2
  Three-Phase Breaker33/LConn3 -- Three-Phase Transformer (Two Windings)2/RConn3
  Three-Phase Breaker35/LConn1 -- Three-Phase Transformer (Two Windings)7/RConn1
  Three-Phase Breaker35/LConn2 -- Three-Phase Transformer (Two Windings)7/RConn2
  Three-Phase Breaker35/LConn3 -- Three-Phase Transformer (Two Windings)7/RConn3
  Three-Phase Breaker36/LConn1 -- Three-Phase Transformer (Two Windings)8/RConn1
  Three-Phase Breaker36/LConn2 -- Three-Phase Transformer (Two Windings)8/RConn2
  Three-Phase Breaker36/LConn3 -- Three-Phase Transformer (Two Windings)8/RConn3
  Three-Phase Transformer (Two Windings)9/LConn2 -- Three-Phase Breaker38/RConn2
  Three-Phase Transformer (Two Windings)9/LConn1 -- Three-Phase Breaker38/RConn1
  Three-Phase Transformer (Two Windings)9/LConn3 -- Three-Phase Breaker38/RConn3
  Three-Phase Transformer (Two Windings)11/RConn1 -- Three-Phase Breaker1/LConn1
  Three-Phase Breaker1/LConn2 -- Three-Phase Transformer (Two Windings)11/RConn2
  Three-Phase Breaker1/LConn3 -- Three-Phase Transformer (Two Windings)11/RConn3
  Three-Phase Transformer (Two Windings)11/LConn1 -- Three-Phase Breaker37/LConn1
  Three-Phase Transformer (Two Windings)11/LConn2 -- Three-Phase Breaker37/LConn2
  Three-Phase Transformer (Two Windings)11/LConn3 -- Three-Phase Breaker37/LConn3
  Three-Phase Breaker39/LConn1 -- Three-Phase Series RLC Load11/LConn1
  Three-Phase Breaker39/LConn2 -- Three-Phase Series RLC Load11/LConn2
  Three-Phase Breaker39/LConn3 -- Three-Phase Series RLC Load11/LConn3
  Three-Phase Breaker40/LConn1 -- Three-Phase Series RLC Load12/LConn1
  Three-Phase Breaker40/LConn2 -- Three-Phase Series RLC Load12/LConn2
  Three-Phase Breaker40/LConn3 -- Three-Phase Series RLC Load12/LConn3
  Three-Phase Series RLC Load3/LConn1 -- Three-Phase Breaker12/RConn1
  Three-Phase Series RLC Load3/LConn3 -- Three-Phase Breaker12/RConn3
  Three-Phase Series RLC Load3/LConn2 -- Three-Phase Breaker12/RConn2
  Three-Phase Series RLC Load14/LConn3 -- Three-Phase Breaker41/RConn3
  Three-Phase Series RLC Load14/LConn1 -- Three-Phase Breaker41/RConn1
  Three-Phase Series RLC Load14/LConn2 -- Three-Phase Breaker41/RConn2
  Three-Phase Breaker12/LConn1 -- Three-Phase Breaker41/LConn1 -- Three-Phase Transformer (Two Windings)8/LConn1
  Three-Phase Breaker12/LConn2 -- Three-Phase Breaker41/LConn2 -- Three-Phase Transformer (Two Windings)8/LConn2
  Three-Phase Breaker12/LConn3 -- Three-Phase Breaker41/LConn3 -- Three-Phase Transformer (Two Windings)8/LConn3
  Three-Phase Series RLC Load13/LConn3 -- Three-Phase Breaker11/RConn3
  Three-Phase Series RLC Load13/LConn1 -- Three-Phase Breaker11/RConn1
  Three-Phase Series RLC Load13/LConn2 -- Three-Phase Breaker11/RConn2
  Three-Phase Series RLC Load1/LConn1 -- Three-Phase Breaker1/RConn1
  Three-Phase Series RLC Load1/LConn3 -- Three-Phase Breaker1/RConn3
  Three-Phase Series RLC Load1/LConn2 -- Three-Phase Breaker1/RConn2
  Three-Phase Transformer (Two Windings)3/LConn1 -- Three-Phase Breaker32/LConn1
  Three-Phase Transformer (Two Windings)3/LConn2 -- Three-Phase Breaker32/LConn2
  Three-Phase Transformer (Two Windings)3/LConn3 -- Three-Phase Breaker32/LConn3
  Three-Phase Transformer (Two Windings)3/RConn1 -- Three-Phase Breaker4/RConn1
  Three-Phase Breaker4/RConn3 -- Three-Phase Transformer (Two Windings)3/RConn3
  Three-Phase Breaker4/RConn2 -- Three-Phase Transformer (Two Windings)3/RConn2
  Three-Phase Breaker13/RConn1 -- Three-Phase Transformer (Two Windings)7/LConn1
  Three-Phase Breaker13/RConn2 -- Three-Phase Transformer (Two Windings)7/LConn2
  Three-Phase Breaker13/RConn3 -- Three-Phase Transformer (Two Windings)7/LConn3
  Three-Phase Breaker13/LConn1 -- Three-Phase Series RLC Load4/LConn1
  Three-Phase Breaker13/LConn2 -- Three-Phase Series RLC Load4/LConn2
  Three-Phase Breaker13/LConn3 -- Three-Phase Series RLC Load4/LConn3
  Three-Phase Transformer (Two Windings)1/RConn1 -- Three-Phase Breaker34/LConn1
  Three-Phase Transformer (Two Windings)1/RConn2 -- Three-Phase Breaker34/LConn2
  Three-Phase Transformer (Two Windings)1/RConn3 -- Three-Phase Breaker34/LConn3
